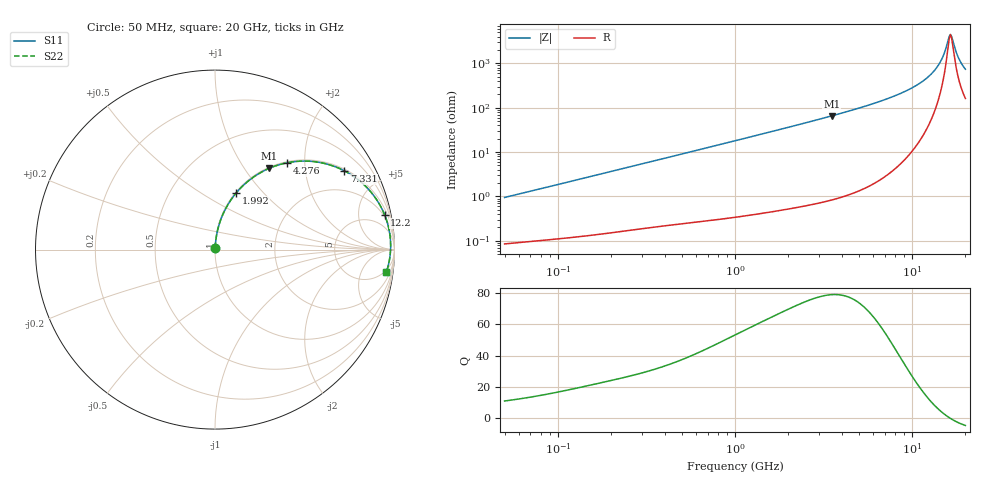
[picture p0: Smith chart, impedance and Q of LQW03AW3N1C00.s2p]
!Murata Part Number: LQW03AW3N1C00
!These Parameters are Measured in Series Mode Connection
!  o--[Z]--o
!Port1  Port2
!  o-------o
!Freq. Start=50[MHz] Stop=20[GHz], 401[Steps]
# Hz S RI R 50
!Freq.(Hz) S11(Real) S11(Imag) S21(Real) S21(Imag) S12(Real) S12(Imag) S22(Real) S22(Imag)
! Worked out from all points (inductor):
!   401 points, 50 MHz to 20 GHz, reference 50 ohm
!   read as one part in series: L = 2.99 nH near 51.52 MHz
!   highest Q = 78.8 at 3.519 GHz (marker M1), where L = 2.97 nH
!   self-resonance near 16.46 GHz
!   S11 on the Smith chart (normalised r, x): 50 MHz: 1.00, +0.02; 1.992 GHz: 1.01, +0.72; 4.276 GHz: 1.02, +1.63; 7.331 GHz: 1.06, +3.25; 12.2 GHz: 1.71, +9.54; 20 GHz: 4, -14
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5e7  0.00094 0.00945  0.9991 -0.00945  0.9991 -0.00945  0.00094 0.00945
1.364002e8  0.00189 0.0251  0.9981 -0.0251  0.9981 -0.0251  0.00189 0.0251
3.721004e8  0.00661 0.067  0.9934 -0.067  0.9934 -0.067  0.00661 0.067
1e9  0.0345 0.1732  0.9655 -0.1732  0.9655 -0.1732  0.0345 0.1732
1.99176e9  0.1187 0.3163  0.8813 -0.3163  0.8813 -0.3163  0.1187 0.3163
2.728004e9  0.203 0.3957  0.797 -0.3957  0.797 -0.3957  0.203 0.3957
3.519108e9  0.3033 0.4534  0.6967 -0.4534  0.6967 -0.4534  0.3033 0.4534
4.275624e9  0.4006 0.4836  0.5994 -0.4836  0.5994 -0.4836  0.4006 0.4836
5.683258e9  0.567 0.4882  0.433 -0.4882  0.433 -0.4882  0.567 0.4882
7.331367e9  0.7213 0.4387  0.2787 -0.4387  0.2787 -0.4387  0.7213 0.4387
7.442007e9  0.73 0.4341  0.27 -0.4341  0.27 -0.4341  0.73 0.4341
9.892087e9  0.8743 0.3139  0.1257 -0.3139  0.1257 -0.3139  0.8743 0.3139
1.220001e10  0.9449 0.1939  0.0551 -0.1939  0.0551 -0.1939  0.9449 0.1939
1.334722e10  0.9636 0.1374  0.0364 -0.1374  0.0364 -0.1374  0.9636 0.1374
1.438523e10  0.9735 0.0891  0.0265 -0.0891  0.0265 -0.0891  0.9735 0.0891
1.504638e10  0.977 0.0597  0.023 -0.0597  0.023 -0.0597  0.977 0.0597
1.597544e10  0.9786 0.0206  0.0214 -0.0206  0.0214 -0.0206  0.9786 0.0206
1.646126e10  0.9782 0.00101  0.0218 -0.00101  0.0218 -0.00101  0.9782 0.00101
1.696185e10  0.977 -0.0185  0.023 0.0185  0.023 0.0185  0.977 -0.0185
1.774144e10  0.9735 -0.0474  0.0265 0.0474  0.0265 0.0474  0.9735 -0.0474
1.855685e10  0.9682 -0.076  0.0318 0.076  0.0318 0.076  0.9682 -0.076
2e10  0.9555 -0.1226  0.0445 0.1226  0.0445 0.1226  0.9555 -0.1226
